TYPE VAT_OUT :
STRUCT
	Target_Pressure	:	REAL	;
	Target_Position	:	REAL	;
	Pressure_Input_Digital_Sensor_1	:	REAL	;
	Pressure_Input_Digital_Sensor_2	:	REAL	;
	Control_Mode	:	SINT	;						(*	0 = init 
															1 = homing 
															2 = position 
															3 = close 
															4 = open 
															5 = pressure 
															6 = hold 
															7 = learn 
															8 = interlock open 
															9 = interlock close 
															12 = power failure 
															13 = safety 
															14 = fatal error
														*)
	General_Control_Setpoint	:	UINT	;
	Pressure_Ramp_Time	:	REAL	;
	Controller_Sel		:	USINT;
	Bank_Sel			:	USINT;
END_STRUCT
END_TYPE
